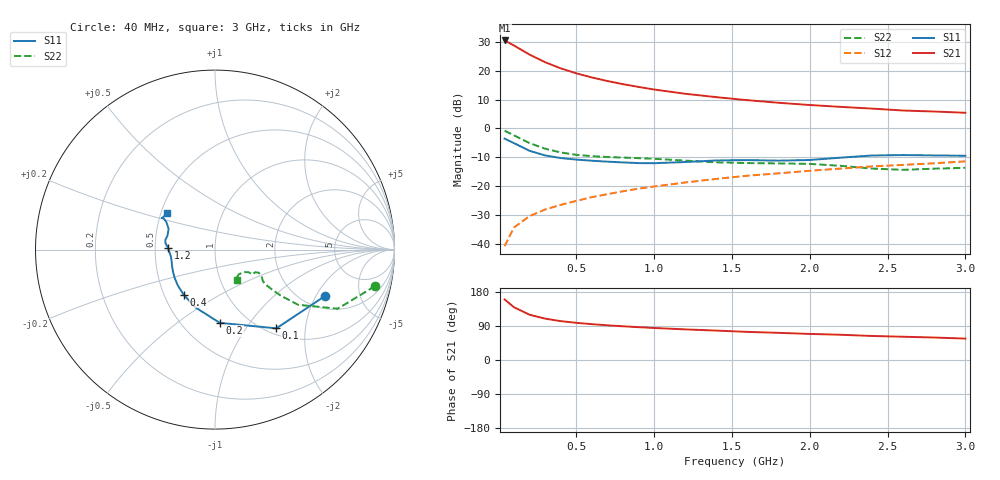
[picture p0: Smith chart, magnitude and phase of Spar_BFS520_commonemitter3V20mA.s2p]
! Filename:  BFS520E.S2P  Version:  4.0
! NXP part #: BFS520  Date: Jun 1994
! Bias condition: Vce=3V, Ic=20mA
#  MHz  S  MA  R  50
! Freq  S11  S21  S12  S22  !GUM [dB]
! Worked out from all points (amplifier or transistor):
!   21 points, 40 MHz to 3 GHz, reference 50 ohm
!   highest |S21| = 30.6 dB at 40 MHz (marker M1)
!   |S21| within 3 dB of that: start of sweep to 139.5 MHz
!   unconditionally stable (mu >= 1): 614.9 MHz to end of sweep
!   at 300 MHz: K = 0.81, MSG = 25.6 dB, |S12| = -28.2 dB
!   at 1 GHz: K = 1.08, MAG = 15.2 dB, |S12| = -20.2 dB
!   at 3 GHz: K = 1.04, MAG = 7.2 dB, |S12| = -11.4 dB
!   lowest NFmin = 1.45 dB at 500 MHz
!   S11 on the Smith chart (normalised r, x): 40 MHz: 2.57, -2.38; 100 MHz: 1.10, -1.40; 200 MHz: 0.75, -0.73; 400 MHz: 0.63, -0.35; 1.2 GHz: 0.59, +0.01; 3 GHz: 0.54, +0.25
40  0.665 -22.9  33.84 159.8  0.009 80.4  0.914 -12.9
100  0.556 -52.1  27.65 139.3  0.019 69.1  0.759 -25.7
200  0.409 -86.3  19.23 119.5  0.03 63.7  0.556 -33.6
300  0.34 -108.7  14.18 109.2  0.039 64.7  0.445 -35.0
400  0.306 -124.8  11.09 102.6  0.047 66.4  0.383 -35.0
500  0.288 -135.9  9.094 98.1  0.055 68.1  0.348 -34.6
600  0.275 -144.5  7.701 94.6  0.064 69.6  0.33 -34.0
700  0.265 -151.9  6.681 91.6  0.072 70.9  0.319 -33.3
800  0.257 -158.4  5.888 89.0  0.081 71.7  0.312 -32.1
900  0.25 -165.1  5.266 86.6  0.09 72.2  0.305 -30.8
1000  0.249 -171.4  4.754 84.5  0.098 72.7  0.297 -29.6
1200  0.261 178.3  4.007 80.8  0.115 73.3  0.276 -27.9
1400  0.278 172.7  3.501 77.6  0.133 73.8  0.258 -29.2
1600  0.282 169.1  3.1 74.2  0.151 73.2  0.25 -32.9
1800  0.276 164.0  2.794 71.7  0.166 73.4  0.247 -34.0
2000  0.283 155.9  2.557 68.8  0.184 72.9  0.242 -33.6
2200  0.311 150.5  2.37 66.6  0.201 72.9  0.224 -34.1
2400  0.339 148.5  2.215 63.4  0.219 72.4  0.201 -38.7
2600  0.345 149.4  2.05 61.4  0.233 71.3  0.191 -47.0
2800  0.34 147.7  1.97 59.3  0.248 71.3  0.2 -52.8
3000  0.335 142.2  1.873 56.5  0.268 70.6  0.207 -54.5
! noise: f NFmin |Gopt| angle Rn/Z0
500  1.45  0.048  61  0.2
900  1.6  0.078  136  0.18
2000  2.2  0.311  -153  0.17
